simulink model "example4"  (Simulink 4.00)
settings: Solver=ode45  StartTime=0.0  StopTime=20.0  RelTol=1e-3

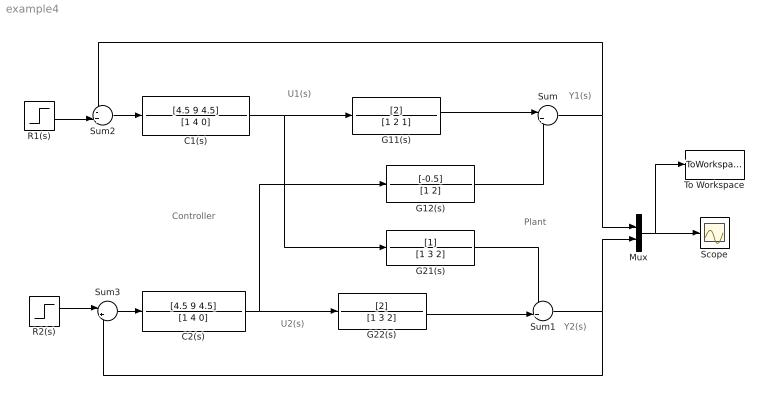
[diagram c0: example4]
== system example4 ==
  note: Y1(s)
  note: Y2(s)
  note: U1(s)
  note: U2(s)
  note: Plant
  note: Controller
  C1(s) : TransferFcn  Numerator=[4.5 9 4.5]  Denominator=[1 4 0]  AbsoluteTolerance=auto  Realization=auto
  C2(s) : TransferFcn  Numerator=[4.5 9 4.5]  Denominator=[1 4 0]  AbsoluteTolerance=auto  Realization=auto
  G11(s) : TransferFcn  Numerator=[2]  Denominator=[1 2 1]  AbsoluteTolerance=auto  Realization=auto
  G12(s) : TransferFcn  Numerator=[-0.5]  Denominator=[1 2]  AbsoluteTolerance=auto  Realization=auto
  G21(s) : TransferFcn  Numerator=[1]  Denominator=[1 3 2]  AbsoluteTolerance=auto  Realization=auto
  G22(s) : TransferFcn  Numerator=[2]  Denominator=[1 3 2]  AbsoluteTolerance=auto  Realization=auto
  Mux : Mux  Inputs=2
  R1(s) : Step  Time=1  Before=0  After=1  SampleTime=0
  R2(s) : Step  Time=5  Before=0  After=-1  SampleTime=0
  Scope : Scope
  Sum : Sum  Inputs=|++  SaturateOnIntegerOverflow=on
  Sum1 : Sum  Inputs=++|  SaturateOnIntegerOverflow=on
  Sum2 : Sum  Inputs=-+|  SaturateOnIntegerOverflow=on
  Sum3 : Sum  Inputs=|+-  SaturateOnIntegerOverflow=on
  To Workspace : ToWorkspace  VariableName=Y  SampleTime=-1  SaveFormat=Array
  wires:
  G11(s)/1 -> Sum/1
  Sum/1 -> Mux/1, Sum2/1
  G22(s)/1 -> Sum1/2
  Sum1/1 -> Mux/2, Sum3/2
  G12(s)/1 -> Sum/2
  G21(s)/1 -> Sum1/1
  C1(s)/1 -> G21(s)/1, G11(s)/1
  C2(s)/1 -> G12(s)/1, G22(s)/1
  R1(s)/1 -> Sum2/2
  Sum2/1 -> C1(s)/1
  Sum3/1 -> C2(s)/1
  R2(s)/1 -> Sum3/1
  Mux/1 -> Scope/1, To Workspace/1
